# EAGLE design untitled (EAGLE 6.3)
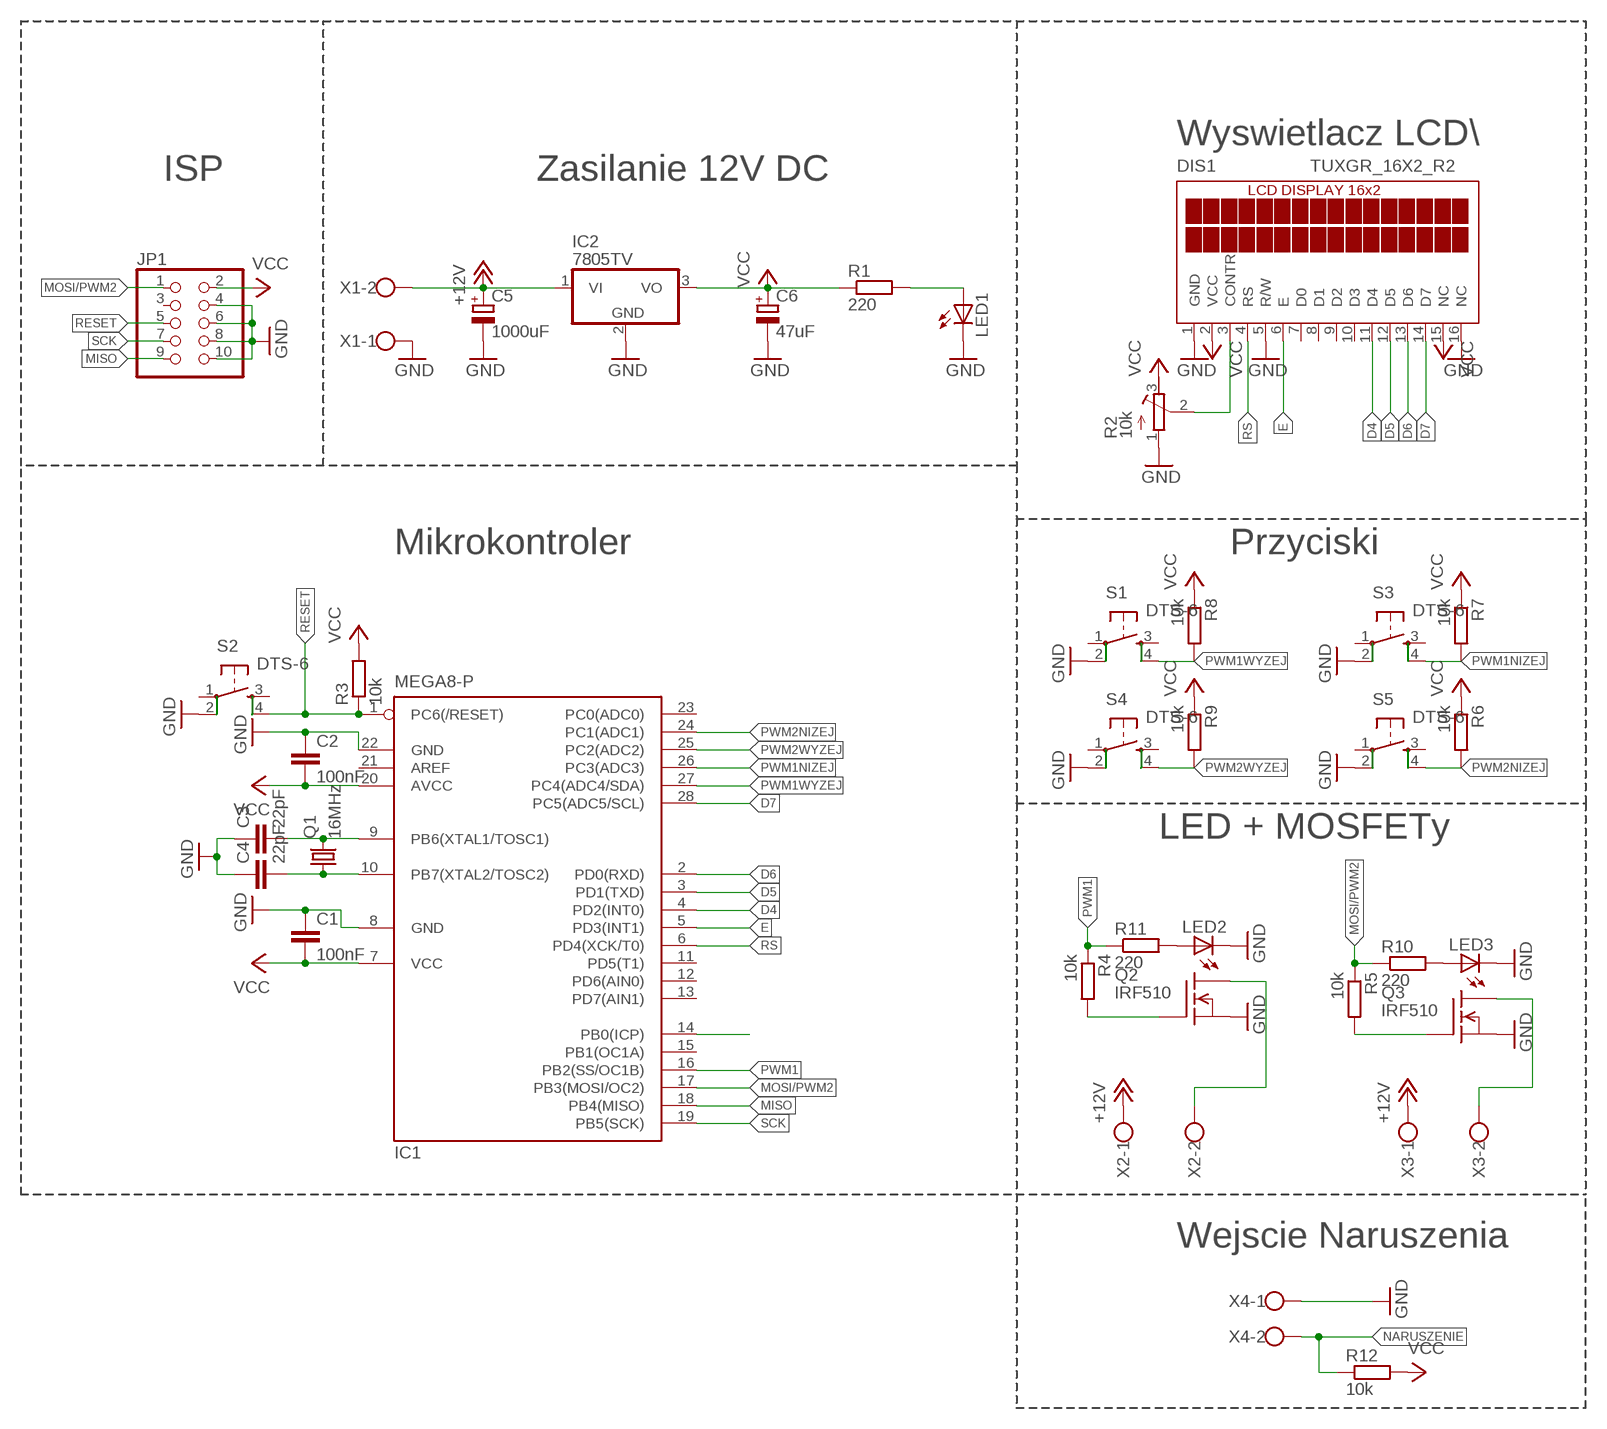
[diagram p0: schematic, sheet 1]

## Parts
C1  100nF  C-EU025-025X050  [C025-025X050]
C2  100nF  C-EU025-025X050  [C025-025X050]
C3  22pF  C-EU025-025X050  [C025-025X050]
C4  22pF  C-EU025-025X050  [C025-025X050]
C5  1000uF  CPOL-EUE3.5-10  [E3,5-10]
C6  47uF  CPOL-EUE2.5-6  [E2,5-6]
DIS1  TUXGR_16X2_R2  [TUXGR_16X2_R2]
IC1  MEGA8-P  [DIL28-3]
IC2  7805TV  [TO220V]
JP1  PINHD-2X5  [2X05]
LED1  LED3MM  [LED3MM]
LED2  LED3MM  [LED3MM]
LED3  LED3MM  [LED3MM]
Q1  16MHz  CRYSTALHC49S  [HC49/S]
Q2  IRF510  [TO220]
Q3  IRF510  [TO220]
R1  220  R-EU_0204/7  [0204/7]
R2  10k  R-TRIMM3339P  [RTRIM3339P]
R3  10k  R-EU_0204/7  [0204/7]
R4  10k  R-EU_0204/7  [0204/7]
R5  10k  R-EU_0204/7  [0204/7]
R6  10k  R-EU_0204/7  [0204/7]
R7  10k  R-EU_0204/7  [0204/7]
R8  10k  R-EU_0204/7  [0204/7]
R9  10k  R-EU_0204/7  [0204/7]
R10  220  R-EU_0204/7  [0204/7]
R11  220  R-EU_0204/7  [0204/7]
R12  10k  R-EU_0204/7  [0204/7]
S1  DTS-6  [DTS-6]
S2  DTS-6  [DTS-6]
S3  DTS-6  [DTS-6]
S4  DTS-6  [DTS-6]
S5  DTS-6  [DTS-6]
X1  W237-102  [W237-102]
X2  W237-113  [W237-113]
X3  W237-113  [W237-113]
X4  W237-102  [W237-102]

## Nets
+12V: C5.+ IC2.1(VI) X1.2 X2.1 X3.1
D4: DIS1.11(D4) IC1.4(PD2(INT0))
D5: DIS1.12(D5) IC1.3(PD1(TXD))
D6: DIS1.13(D6) IC1.2(PD0(RXD))
D7: DIS1.14(D7) IC1.28(PC5(ADC5/SCL))
E: DIS1.6(E) IC1.5(PD3(INT1))
GND: C1.1 C2.1 C3.1 C4.1 C5.- C6.- DIS1.1(GND) DIS1.5(R/W) DIS1.16(NC) IC1.8(GND) IC1.22(GND) IC2.2(GND) JP1.4 JP1.6 JP1.8 JP1.10 LED1.K(C) LED2.K(C) LED3.K(C) Q2.3(S) Q3.3(S) R2.1(E) S1.2 S2.2 S3.2 S4.2 S5.2 X1.1 X4.1
MISO: IC1.18(PB4(MISO)) JP1.9
MOSI/PWM2: IC1.17(PB3(MOSI/OC2)) JP1.1 R5.1 R10.1
N$1: Q2.1(G) R4.2
N$2: Q3.1(G) R5.2
N$3: LED1.A R1.2
N$4: DIS1.3(CONTR) R2.2(S)
N$5: Q2.2(D) X2.2
N$6: Q3.2(D) X3.2
N$7: LED2.A R11.2
N$8: LED3.A R10.2
N$14: C4.2 IC1.10(PB7(XTAL2/TOSC2)) Q1.1
N$15: C3.2 IC1.9(PB6(XTAL1/TOSC1)) Q1.2
NARUSZENIE: IC1.14(PB0(ICP)) R12.1 X4.2
PWM1: IC1.16(PB2(SS/OC1B)) R4.1 R11.1
PWM1NIZEJ: IC1.26(PC3(ADC3)) R7.2 S3.4
PWM1WYZEJ: IC1.27(PC4(ADC4/SDA)) R8.2 S1.4
PWM2NIZEJ: IC1.24(PC1(ADC1)) R6.2 S5.4
PWM2WYZEJ: IC1.25(PC2(ADC2)) R9.2 S4.4
RESET: IC1.1(PC6(/RESET)) JP1.5 R3.1 S2.4
RS: DIS1.4(RS) IC1.6(PD4(XCK/T0))
SCK: IC1.19(PB5(SCK)) JP1.7
VCC: C1.2 C2.2 C6.+ DIS1.2(VCC) DIS1.15(NC) IC1.7(VCC) IC1.20(AVCC) IC2.3(VO) JP1.2 R1.1 R2.3(A) R3.2 R6.1 R7.1 R8.1 R9.1 R12.2
Unconnected: DIS1.7(D0) DIS1.8(D1) DIS1.9(D2) DIS1.10(D3) IC1.11(PD5(T1)) IC1.12(PD6(AIN0)) IC1.13(PD7(AIN1)) IC1.15(PB1(OC1A)) IC1.21(AREF) IC1.23(PC0(ADC0)) JP1.3 S1.1 S1.3 S2.1 S2.3 S3.1 S3.3 S4.1 S4.3 S5.1 S5.3

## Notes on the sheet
- Wyswietlacz LCD\
- ISP | Zasilanie 12V DC
- Mikrokontroler | Przyciski
- LED + MOSFETy
- Wejscie Naruszenia

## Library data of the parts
C1-C4 = resistor:C-EU: CAPACITOR, European symbol
C5 C6 = resistor:CPOL-EU: POLARIZED CAPACITOR, European symbol
DIS1 = display-lcd:TUXGR_16X2_R2: Tuxgraphics LCD display 16x2 characters reflective, without background light Source: tuxgr_12x2_r2.pdf; OC_FARNELL: unknown; OC_NEWARK: unknown
IC1 = atmel:MEGA8-P: MICROCONTROLLER 8 Kbytes FLASH, 1 kbytes SRAM, 512 bytes EEPROM, USART, 4-channel 10 bit ADC, 2-channel 8 bit ADC Pin compatible with Atmega48, ATMega88, ATMega168 Source: avr.lbr
IC2 = linear:78*: Positive VOLTAGE REGULATOR Source: http://cache.national.com/ds/LM/LM78L05.pdf http://www.fairchildsemi.com/ds/LM/LM7805.pdf
JP1 = pinhead:PINHD-2X5: PIN HEADER
LED1-LED3 = led:LED: LED
Q1 = crystal:CRYSTAL: CRYSTAL; OC_FARNELL: 1667008; OC_NEWARK: unknown
Q2 Q3 = transistor-fet:IRF510: N-Channel Enhancement MOSFET (HEXFET); 100V; 5,6A; 0,54Ohm
R1 R3-R12 = resistor:R-EU_: RESISTOR, European symbol
R2 = resistor:R-TRIMM: Trimm resistor
S1-S5 = switch-tact:DTS-6
X1 X4 = con-wago-500:W237-102: WAGO SCREW CLAMP; MPN: 237-102; OC_FARNELL: unknown; OC_NEWARK: 70K9898
X2 X3 = con-wago-500:W237-113: WAGO SCREW CLAMP; OC_FARNELL: unknown; OC_NEWARK: unknown

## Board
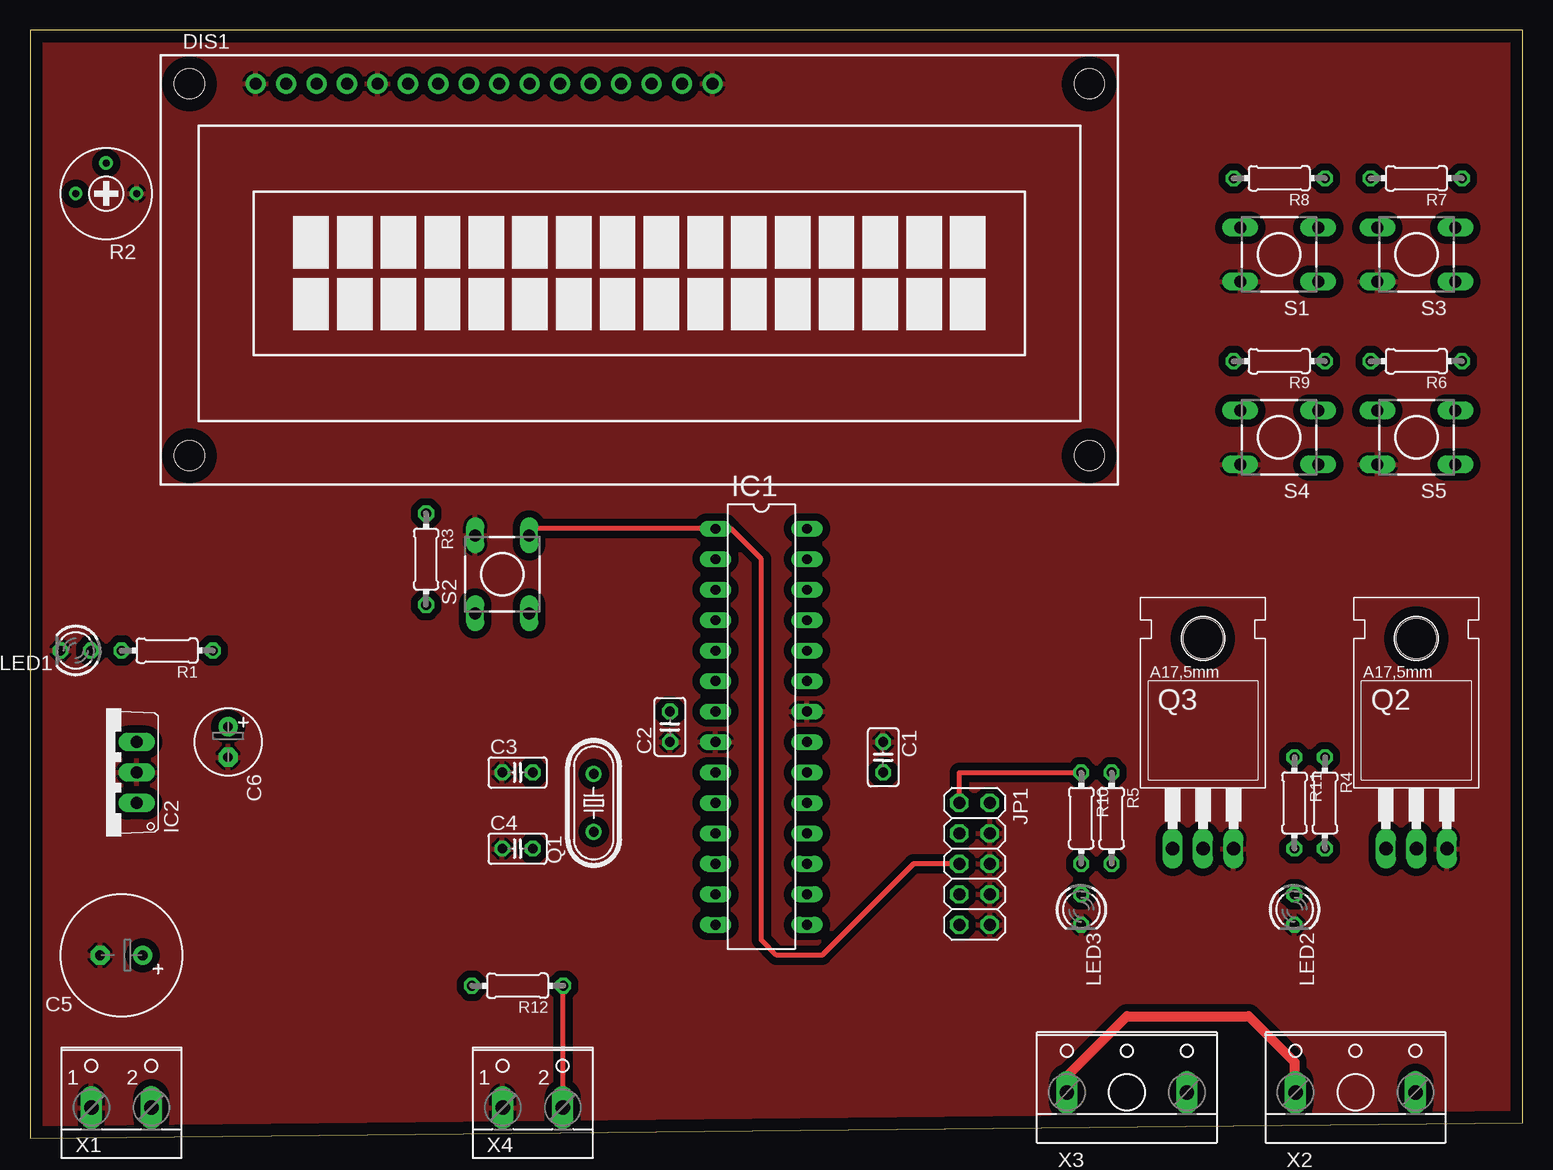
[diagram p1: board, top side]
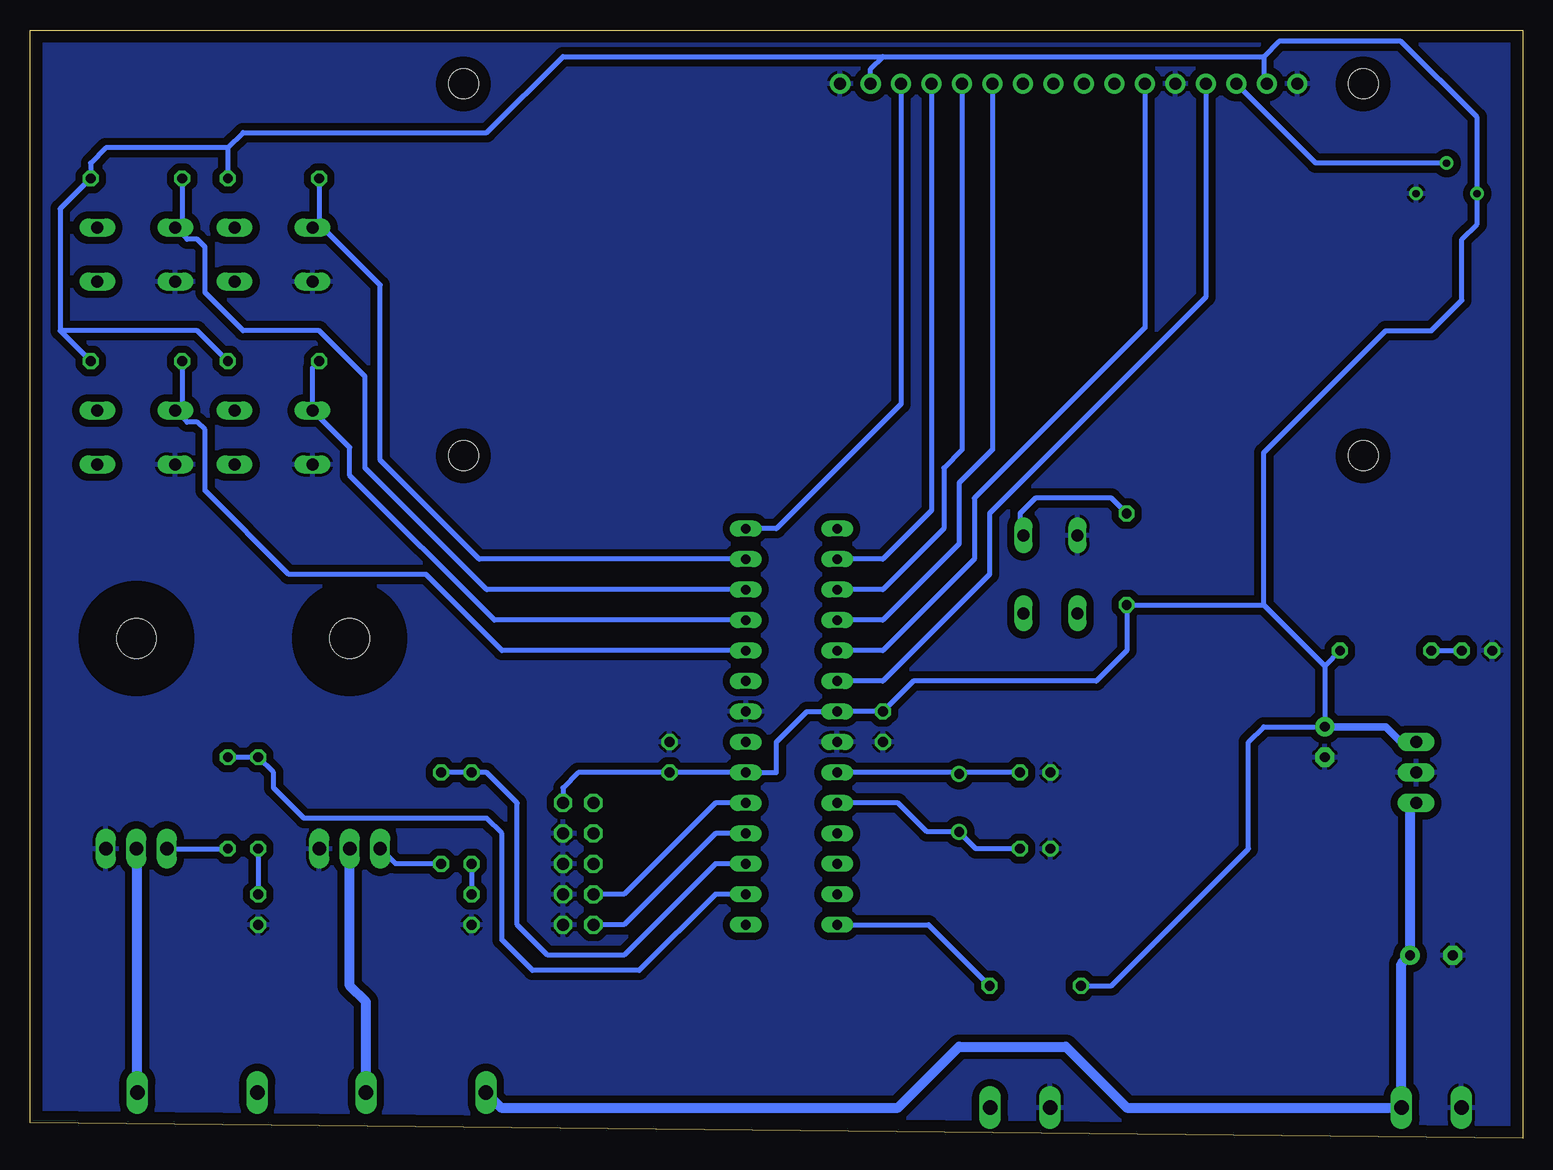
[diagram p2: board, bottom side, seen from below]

Size 124.44 x 92.38 mm. Coordinates in mm from the lower left corner, seen from the top.
Outline: 0,0 124.44,1.27 124.44,92.38 0,92.38 0,0
Copper layers (1*16): Top 0.035mm / dielectric 1.5mm / Bottom 0.035mm
Design rules "default": minimum track width 10mil, minimum drill 24mil, track to track 8mil, track to pad 8mil, pad to pad 8mil, via to via 8mil, smd to smd 8mil, copper to edge 40mil, drill to drill 8mil, minimum pad ring 10mil, minimum via ring 8mil, stop-mask expansion 4mil, vias tented up to drill 0mil, thermal gap 10mil

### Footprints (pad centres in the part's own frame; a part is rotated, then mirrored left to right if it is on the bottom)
C025-025X050 = drill 0.813 octagon: 1 -1.27,0; 2 1.27,0
E3,5-10 = drill 0.813 pad 1.6: + -1.778,0 | drill 0.813 pad 1.6 octagon: - 1.778,0
E2,5-6 = drill 0.813 pad 1.6: + -1.27,0 | drill 0.813 pad 1.6 octagon: - 1.27,0
TUXGR_16X2_R2 = drill 1 pad 1.676: 1 -32,15.5; 2 -29.46,15.5; 3 -26.92,15.5; 4 -24.38,15.5; 5 -21.84,15.5; 6 -19.3,15.5; 7 -16.76,15.5; 8 -14.22,15.5; 9 -11.68,15.5; 10 -9.14,15.5; 11 -6.6,15.5; 12 -4.06,15.5; 13 -1.52,15.5; 14 1.02,15.5; 15 3.56,15.5; 16 6.1,15.5 | hole 2.5: -37.5,-15.5; 37.5,-15.5; -37.5,15.5; 37.5,15.5
DIL28-3 = drill 0.813 long: 1 -16.51,-3.81; 2 -13.97,-3.81; 3 -11.43,-3.81; 4 -8.89,-3.81; 5 -6.35,-3.81; 6 -3.81,-3.81; 7 -1.27,-3.81; 8 1.27,-3.81; 9 3.81,-3.81; 10 6.35,-3.81; 11 8.89,-3.81; 12 11.43,-3.81; 13 13.97,-3.81; 14 16.51,-3.81; 15 16.51,3.81; 16 13.97,3.81; 17 11.43,3.81; 18 8.89,3.81; 19 6.35,3.81; 20 3.81,3.81; 21 1.27,3.81; 22 -1.27,3.81; 23 -3.81,3.81; 24 -6.35,3.81; 25 -8.89,3.81; 26 -11.43,3.81; 27 -13.97,3.81; 28 -16.51,3.81
TO220V = drill 1.016 long: 1 -2.54,-2.54; 2 0,-2.54; 3 2.54,-2.54
2X05 = drill 1.016 octagon: 1 -5.08,-1.27; 2 -5.08,1.27; 3 -2.54,-1.27; 4 -2.54,1.27; 5 0,-1.27; 6 0,1.27; 7 2.54,-1.27; 8 2.54,1.27; 9 5.08,-1.27; 10 5.08,1.27
LED3MM = drill 0.813 octagon: A -1.27,0; K 1.27,0
HC49/S = drill 0.813: 1 -2.413,0; 2 2.413,0
TO220 = drill 1.118 long: 1 -2.54,-6.35; 2 0,-6.35; 3 2.54,-6.35 | hole 3.302: 0,11.176
0204/7 = drill 0.813 octagon: 1 -3.81,0; 2 3.81,0
RTRIM3339P = drill 0.61: 1 -2.54,0; 2 0,-2.54; 3 2.54,0
DTS-6 = drill 1 long: 1 -3.25,2.25; 2 3.25,2.25; 3 -3.25,-2.25; 4 3.25,-2.25
W237-102 = drill 1.194 long: 1 -2.5,-1.27; 2 2.5,-1.27
W237-113 = drill 1.194 long: 1 -5,-1.27; 2 5,-1.27

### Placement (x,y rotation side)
C1  71.12,31.75 270 top
C2  53.34,34.29 90 top
C3  40.64,30.48 0 top
C4  40.64,24.13 0 top
C5  7.62,15.24 180 top
C6  16.51,33.02 270 top
DIS1  50.8,72.39 0 top
IC1  60.96,34.29 270 top
IC2  6.35,30.48 90 top
JP1  78.74,22.86 270 top
LED1  3.81,40.64 180 top
LED2  105.41,19.05 270 top
LED3  87.63,19.05 270 top
Q1  46.99,27.94 90 top
Q2  115.57,30.48 0 top
Q3  97.79,30.48 0 top
R1  11.43,40.64 180 top
R2  6.35,78.74 180 top
R3  33.02,48.26 270 top
R4  107.95,27.94 270 top
R5  90.17,26.67 270 top
R6  115.57,64.77 180 top
R7  115.57,80.01 180 top
R8  104.14,80.01 180 top
R9  104.14,64.77 180 top
R10  87.63,26.67 270 top
R11  105.41,27.94 270 top
R12  40.64,12.7 180 top
S1  104.14,73.66 180 top
S2  39.37,46.99 90 top
S3  115.57,73.66 180 top
S4  104.14,58.42 180 top
S5  115.57,58.42 180 top
X1  7.62,3.81 0 top
X2  110.49,5.08 0 top
X3  91.44,5.08 0 top
X4  41.91,3.81 0 top

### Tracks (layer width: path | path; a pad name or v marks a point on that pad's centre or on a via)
+12V
  Top 0.813: X3.1 86.44,5.16 91.44,10.16 101.6,10.16 105.41,6.35 105.41,3.89 X2.1
  Bottom 0.813: IC2.1 9.4,27.43 C5.+ 10.12,14.52 X1.2 33.02,2.54 38.1,7.62 46.99,7.62 52.07,2.54 85.17,2.54 X3.1
D4
  Bottom 0.406: DIS1.11 44.2,57.4 46.99,54.61 46.99,49.53 53.34,43.18 IC1.4
D5
  Bottom 0.406: DIS1.12 46.74,57.4 48.26,55.88 48.26,50.8 53.34,45.72 IC1.3
D6
  Bottom 0.406: DIS1.13 49.28,52.32 53.34,48.26 IC1.2
D7
  Bottom 0.406: DIS1.14 51.82,61.21 62.23,50.8 IC1.28
E
  Bottom 0.406: DIS1.6 31.5,67.56 45.72,53.34 45.72,48.26 53.34,40.64 IC1.5
GND
  pour Bottom (isolate 0.61): -5.08,96.52 129.54,96.52 129.54,-6.35 -5.08,-6.35
  pour Top (isolate 0.61): -3.81,96.52 128.27,96.52 128.27,-6.35 -3.81,-6.35
MISO
  Bottom 0.406: IC1.18 67.31,25.4 74.93,17.78 JP1.9
MOSI/PWM2
  Top 0.406: JP1.1 77.47,30.48 R10.1
  Bottom 0.406: IC1.17 67.31,22.86 74.93,15.24 81.28,15.24 83.82,17.78 83.82,27.94 86.36,30.48 R10.1 R5.1
N$1
  Bottom 0.406: Q2.1 R4.2
N$2
  Bottom 0.406: R5.2 93.98,22.86 Q3.1
N$3
  Bottom 0.406: R1.2 LED1.A
N$4
  Bottom 0.406: R2.2 17.27,81.28 DIS1.3
N$5
  Bottom 0.813: X2.2 115.49,24.05 Q2.2
N$6
  Bottom 0.813: X3.2 96.44,11.35 97.79,12.7 Q3.2
N$7
  Bottom 0.406: R11.2 LED2.A
N$8
  Bottom 0.406: R10.2 LED3.A
N$14
  Bottom 0.406: C4.2 45.59,24.13 Q1.1 49.66,25.53 52.07,27.94 IC1.10
N$15
  Bottom 0.406: Q1.2 46.86,30.48 C3.2 IC1.9
NARUSZENIE
  Top 0.406: X4.2 44.45,2.54 R12.1
  Bottom 0.406: IC1.14 49.53,17.78 R12.1
PWM1
  Bottom 0.406: IC1.16 67.31,20.32 73.66,13.97 82.55,13.97 85.09,16.51 85.09,25.4 86.36,26.67 101.6,26.67 104.14,29.21 104.14,30.48 R11.1 R4.1
PWM1NIZEJ
  Bottom 0.406: IC1.26 86.36,45.72 96.52,55.88 96.52,63.5 100.33,67.31 106.68,67.31 109.86,70.48 109.86,74.3 110.49,74.93 111.34,74.93 S3.4 111.76,76.47 R7.2
PWM1WYZEJ
  Bottom 0.406: R8.2 100.33,76.2 | 100.33,76.2 100.6,76.2 S1.4 | IC1.27 87,48.26 95.25,56.52 95.25,71.12 100.33,76.2
PWM2NIZEJ
  Bottom 0.406: IC1.24 85.09,40.64 91.44,46.99 102.87,46.99 109.86,53.98 109.86,59.05 110.49,59.69 111.34,59.69 S5.4 112.03,60.96 111.76,60.96 R6.2
PWM2WYZEJ
  Bottom 0.406: IC1.25 85.72,43.18 97.79,55.25 97.79,57.57 S4.4 100.89,64.21 R9.2
RESET
  Top 0.406: S2.4 41.91,50.53 41.91,50.8 IC1.1 58.42,50.8 60.96,48.26 60.96,16.51 62.23,15.24 66.04,15.24 73.66,22.86 JP1.5
  Bottom 0.406: R3.1 34.29,53.34 40.64,53.34 41.91,52.07 41.91,50.53 S2.4
RS
  Bottom 0.406: DIS1.4 26.42,70.1 44.45,52.07 44.45,46.99 53.34,38.1 IC1.6
SCK
  Bottom 0.406: IC1.19 67.31,27.94 74.93,20.32 JP1.7
VCC
  Bottom 0.406: R1.1 16.51,39.37 | 16.51,39.37 C6.+ 21.59,34.29 22.86,33.02 22.86,24.13 34.29,12.7 R12.2 | 21.59,44.45 R3.2 33.02,40.64 35.56,38.1 50.8,38.1 C2.2 IC1.7 59.69,35.56 62.23,33.02 62.23,30.48 IC1.20 C1.2 78.74,30.48 80.01,29.21 JP1.2 | 21.59,44.45 16.51,39.37 | 21.59,90.17 20.32,91.44 10.16,91.44 3.81,85.09 R2.3 3.81,76.2 5.08,74.93 5.08,69.85 7.62,67.31 11.43,67.31 21.59,57.15 21.59,44.45 | 21.59,90.17 21.59,88.14 DIS1.2 | DIS1.15 54.36,89.15 53.34,90.17 | 53.34,90.17 21.59,90.17 | 107.95,82.55 106.68,83.82 86.36,83.82 80.01,90.17 53.34,90.17 | 107.95,82.55 118.11,82.55 119.38,81.28 R7.1 121.92,77.47 121.92,67.31 | R9.1 110.49,67.31 121.92,67.31 | R6.1 121.92,67.31 | 107.95,82.55 R8.1
  Bottom 0.61: IC2.3 10.16,33.02 11.43,34.29 C6.+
